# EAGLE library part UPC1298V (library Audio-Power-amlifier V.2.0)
The uPC1298V is an integrated monolithic circuit in a 14-SQL type package designed for use in 50W to 80W class HiFi audio power amplifier applications. This device consists of an input differential amplifier, a predriver circuit, a driver circuit, and an over current protection circuit.
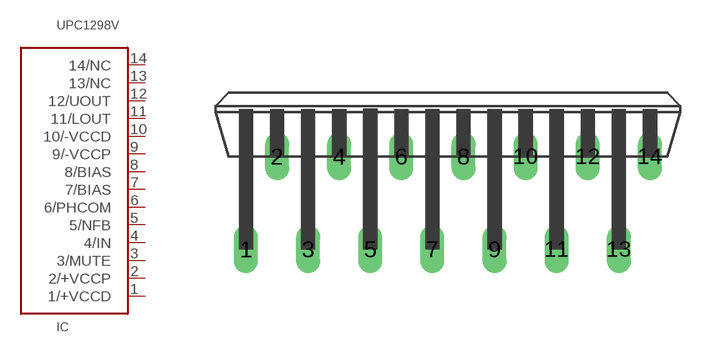
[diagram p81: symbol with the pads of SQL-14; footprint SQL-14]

Designator prefix IC

## UPC1298V  [SQL-14]
1  1/+VCCD  pwr
2  2/+VCCP  pwr
3  3/MUTE
4  4/IN  in
5  5/NFB
6  6/PHCOM
7  7/BIAS
8  8/BIAS
9  9/-VCCP  pwr
10  10/-VCCD  pwr
11  11/LOUT  out
12  12/UOUT  out
13  13/NC  nc
14  14/NC  nc

## Footprint SQL-14 (pad centres in mm)
drill 0.8 long: 1 -11.05,-2.54; 2 -9.35,2.54; 3 -7.65,-2.54; 4 -5.95,2.54; 5 -4.25,-2.54; 6 -2.55,2.54; 7 -0.85,-2.54; 8 0.85,2.54; 9 2.55,-2.54; 10 4.25,2.54; 11 5.95,-2.54; 12 7.65,2.54; 13 9.35,-2.54; 14 11.05,2.54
